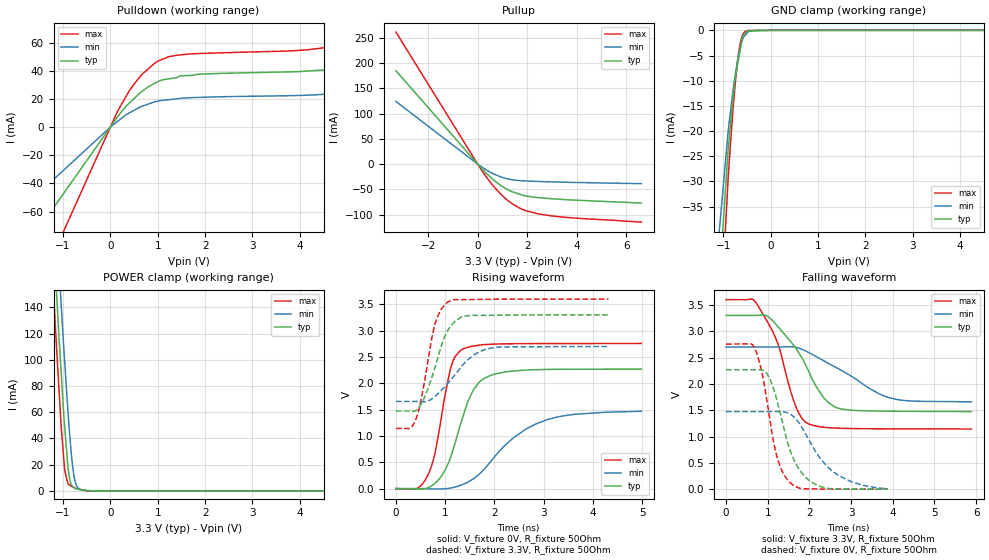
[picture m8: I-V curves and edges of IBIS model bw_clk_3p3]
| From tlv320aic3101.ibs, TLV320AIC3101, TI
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|   bw_clk_3p3 Model
[Model]   bw_clk_3p3
Model_type   I/O
Polarity   Non-Inverting
Enable   Active-Low
Vinl = 0.99
Vinh = 2.31
Vmeas = 1.65
Vref = 1.65
Cref = 2pF
Rref = 50
|   typ   min   max
|   (nom PVT)   (fast PVT)   (slow PVT)
 C_comp   1.335e-12   1.312e-12   1.381e-12
| Where nom  PVT is Nominal Process, 3.3V, 27C
|   Fast PVT is Strong Process,  3.6V, -40C
|   Slow PVT is Weak Process,   2.7V, 105C
[Voltage Range]   3.3   2.7   3.6
|Ambient Temperature   25   85   -40
|Junction Temperature
[Temperature Range]   27   105   -40
[Pullup Reference]   3.3   2.7   3.6
[Pulldown Reference]   0   0   0
[Power Clamp Reference]   3.3   2.7   3.6
[GND Clamp Reference]   0   0   0
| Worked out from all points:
|   slope of the pulldown table from 0 to 0.495 V, typ, clamps not added: 24.6 ohm
|   slope of the pullup table from 0 to 0.495 V, typ, clamps not added: 19.9 ohm
|   GND clamp passes 1 mA (typ) near -0.57 V on its own axis
|   POWER clamp passes 1 mA (typ) near -0.65 V on its own axis
|   falling waveform, V_fixture 3.3V, R_fixture 50Ohm: 20-80 % time 842ps typ, 1.32ns min, 601ps max; typ from 3.3 V to 1.48 V
|   rising waveform, V_fixture 0V, R_fixture 50Ohm: 20-80 % time 492ps typ, 1.02ns min, 330ps max; typ from 0 V to 2.27 V
|   rising waveform, V_fixture 3.3V, R_fixture 50Ohm: 20-80 % time 388ps typ, 595ps min, 292ps max; typ from 1.47 V to 3.3 V
|   falling waveform, V_fixture 0V, R_fixture 50Ohm: 20-80 % time 517ps typ, 812ps min, 384ps max; typ from 2.27 V to 0.002 V
[Pulldown]
|   Voltage   I(typ)   I(min)   I(max)
-3.3V     -157.7mA   -102.3mA   -247.6mA
-132.3mV  -6.322mA   -4.101mA   -9.925mA
154.8mV   7.524mA    4.153mA    11.4mA
385.2mV   16.6mA     9.851mA    25.06mA
684mV     25.82mA    15.04mA    38.01mA
1.008V    32.39mA    18.58mA    47.01mA
1.595V    36.65mA    20.77mA    51.78mA
4.162V    39.88mA    22.75mA    54.99mA
5.145V    44.71mA    26.49mA    62.99mA
5.666V    52.09mA    29.08mA    74.48mA
6.376V    71.49mA    32.59mA    104.3mA
6.6V      80.62mA    33.71mA    118.1mA
[GND Clamp]
|   Voltage   I(typ)   I(min)   I(max)
-3.3V     -1.467A    -1.273A    -1.637A
-1.501V   -109.4mA   -83.9mA    -137.1mA
-897.6mV  -23.81mA   -20.2mA    -29.58mA
-842.4mV  -18.1mA    -15.67mA   -21.85mA
-772.2mV  -11.42mA   -10.53mA   -13.32mA
-745.8mV  -9.26mA    -8.799mA   -10.43mA
-702mV    -6.996mA   -6.224mA   -6.431mA
-622.8mV  -2.9mA     -2.716mA   -1.787mA
-590.7mV  -1.241mA   -1.753mA   -927.4uA
-532.8mV  -546uA     -923.6uA   -190.4uA
-286.2mV  -97.99uA   -2.369uA   -5.611uA
6.6V      0A         0A         0A
[Pullup]
|   Voltage   I(typ)   I(min)   I(max)
-3.3V     185.2mA    124.3mA    261.7mA
136.8mV   -7.535mA   -4.589mA   -10.54mA
633.6mV   -31.13mA   -19.16mA   -43.6mA
939.6mV   -42.5mA    -25.4mA    -59.94mA
1.246V    -51.46mA   -29.66mA   -73.23mA
1.447V    -55.61mA   -31.4mA    -80.33mA
1.861V    -62.28mA   -33.02mA   -90.87mA
2.437V    -66.24mA   -34.26mA   -98.47mA
3.701V    -70.81mA   -36.05mA   -106mA
6.6V      -77.04mA   -38.71mA   -115mA
[POWER Clamp]
|   Voltage   I(typ)   I(min)   I(max)
-3.3V     1.694A     1.712A     1.7A
-1.277V   242.7mA    295.4mA    204.8mA
-1.159V   165.6mA    218.7mA    123.9mA
-1.115V   136.7mA    190mA      96.61mA
-1.037V   89.39mA    141.2mA    48.22mA
-964.8mV  49.13mA    98.77mA    15.96mA
-867.9mV  10.85mA    47.17mA    4.718mA
-801.9mV  3.456mA    20.41mA    3.131mA
-742.5mV  1.951mA    6.907mA    2.13mA
-621mV    753.3uA    885uA      999.2uA
-337.5mV  130.3uA    7.375uA    8.169uA
6.6V      0A         0A         0A
[Ramp]
R_load = 50
|   typ   min   max
dV/dt_r   1.36197/4.90284e-10   0.883856/1.01976e-09   1.65397/3.30089e-10
dV/dt_f   1.0959/8.40487e-10   0.626502/1.31838e-09   1.47417/6.0064e-10
[Falling Waveform]
V_fixture = 3.3V
V_fixture_min = 2.7V
V_fixture_max = 3.6V
R_fixture = 50Ohm
|   Time   V(typ)   V(min)   V(max)
0s        3.3V       2.7V       3.6V
738ps     3.3V       2.7V       3.52V
966ps     3.298V     2.7V       3.216V
1.244ns   3.088V     2.7V       2.761V
1.684ns   2.665V     2.694V     1.551V
1.972ns   2.257V     2.6V       1.243V
2.352ns   1.73V      2.436V     1.176V
2.764ns   1.522V     2.259V     1.157V
3.946ns   1.481V     1.731V     1.146V
5.888ns   1.475V     1.659V     1.144V
[Rising Waveform]
V_fixture = 0V
V_fixture_min = 0V
V_fixture_max = 0V
R_fixture = 50Ohm
|   Time   V(typ)   V(min)   V(max)
0s        1.35nV     20.25nV    793.1pV
418ps     -7.474mV   161.7uV    -269.4uV
640ps     11.93mV    -3.304mV   236.8mV
796ps     103.4mV    -7.568mV   684mV
1.112ns   599.2mV    11.03mV    2.286V
1.358ns   1.359V     78.56mV    2.651V
1.59ns    1.895V     197.7mV    2.711V
1.966ns   2.165V     562.8mV    2.743V
3.052ns   2.263V     1.304V     2.754V
4.986ns   2.269V     1.468V     2.756V
[Rising Waveform]
V_fixture = 3.3V
V_fixture_min = 2.7V
V_fixture_max = 3.6V
R_fixture = 50Ohm
|   Time   V(typ)   V(min)   V(max)
0s        1.473V     1.656V     1.143V
278ps     1.473V     1.656V     1.14V
394ps     1.476V     1.656V     1.292V
512ps     1.606V     1.652V     1.692V
726ps     2.099V     1.701V     2.843V
808ps     2.347V     1.763V     3.17V
1.056ns   3.006V     2.002V     3.544V
1.372ns   3.27V      2.362V     3.589V
1.894ns   3.291V     2.663V     3.596V
4.32ns    3.299V     2.699V     3.6V
[Falling Waveform]
V_fixture = 0V
V_fixture_min = 0V
V_fixture_max = 0V
R_fixture = 50Ohm
|   Time   V(typ)   V(min)   V(max)
0s        2.27V      1.473V     2.757V
682ps     2.27V      1.473V     2.689V
832ps     2.27V      1.473V     2.317V
964ps     2.211V     1.473V     1.758V
1.222ns   1.687V     1.473V     620.8mV
1.356ns   1.264V     1.471V     325.3mV
1.582ns   645.2mV    1.403V     93.99mV
1.986ns   171.8mV    942.4mV    6.822mV
2.536ns   8.881mV    351.1mV    2.968mV
3.88ns    1.968mV    8.561mV    1.001mV
